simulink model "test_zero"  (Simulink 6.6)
settings: Solver=ode45  StartTime=0.0  StopTime=10.0  RelTol=1e-3
libraries: sltpda x3

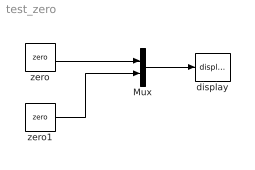
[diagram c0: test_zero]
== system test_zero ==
  Mux : Mux  Inputs=2
  display : sltpda/AO class/display  Tag=display  SystemSampleTime=-1
  zero : sltpda/Modelling/zero  SystemSampleTime=-1  zerof=5  zeroQ=8
  zero1 : sltpda/Modelling/zero  Tag=zero  SystemSampleTime=-1  zerof=6  zeroQ=0
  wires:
  zero1/1 -> Mux/2
  zero/1 -> Mux/1
  Mux/1 -> display/1
